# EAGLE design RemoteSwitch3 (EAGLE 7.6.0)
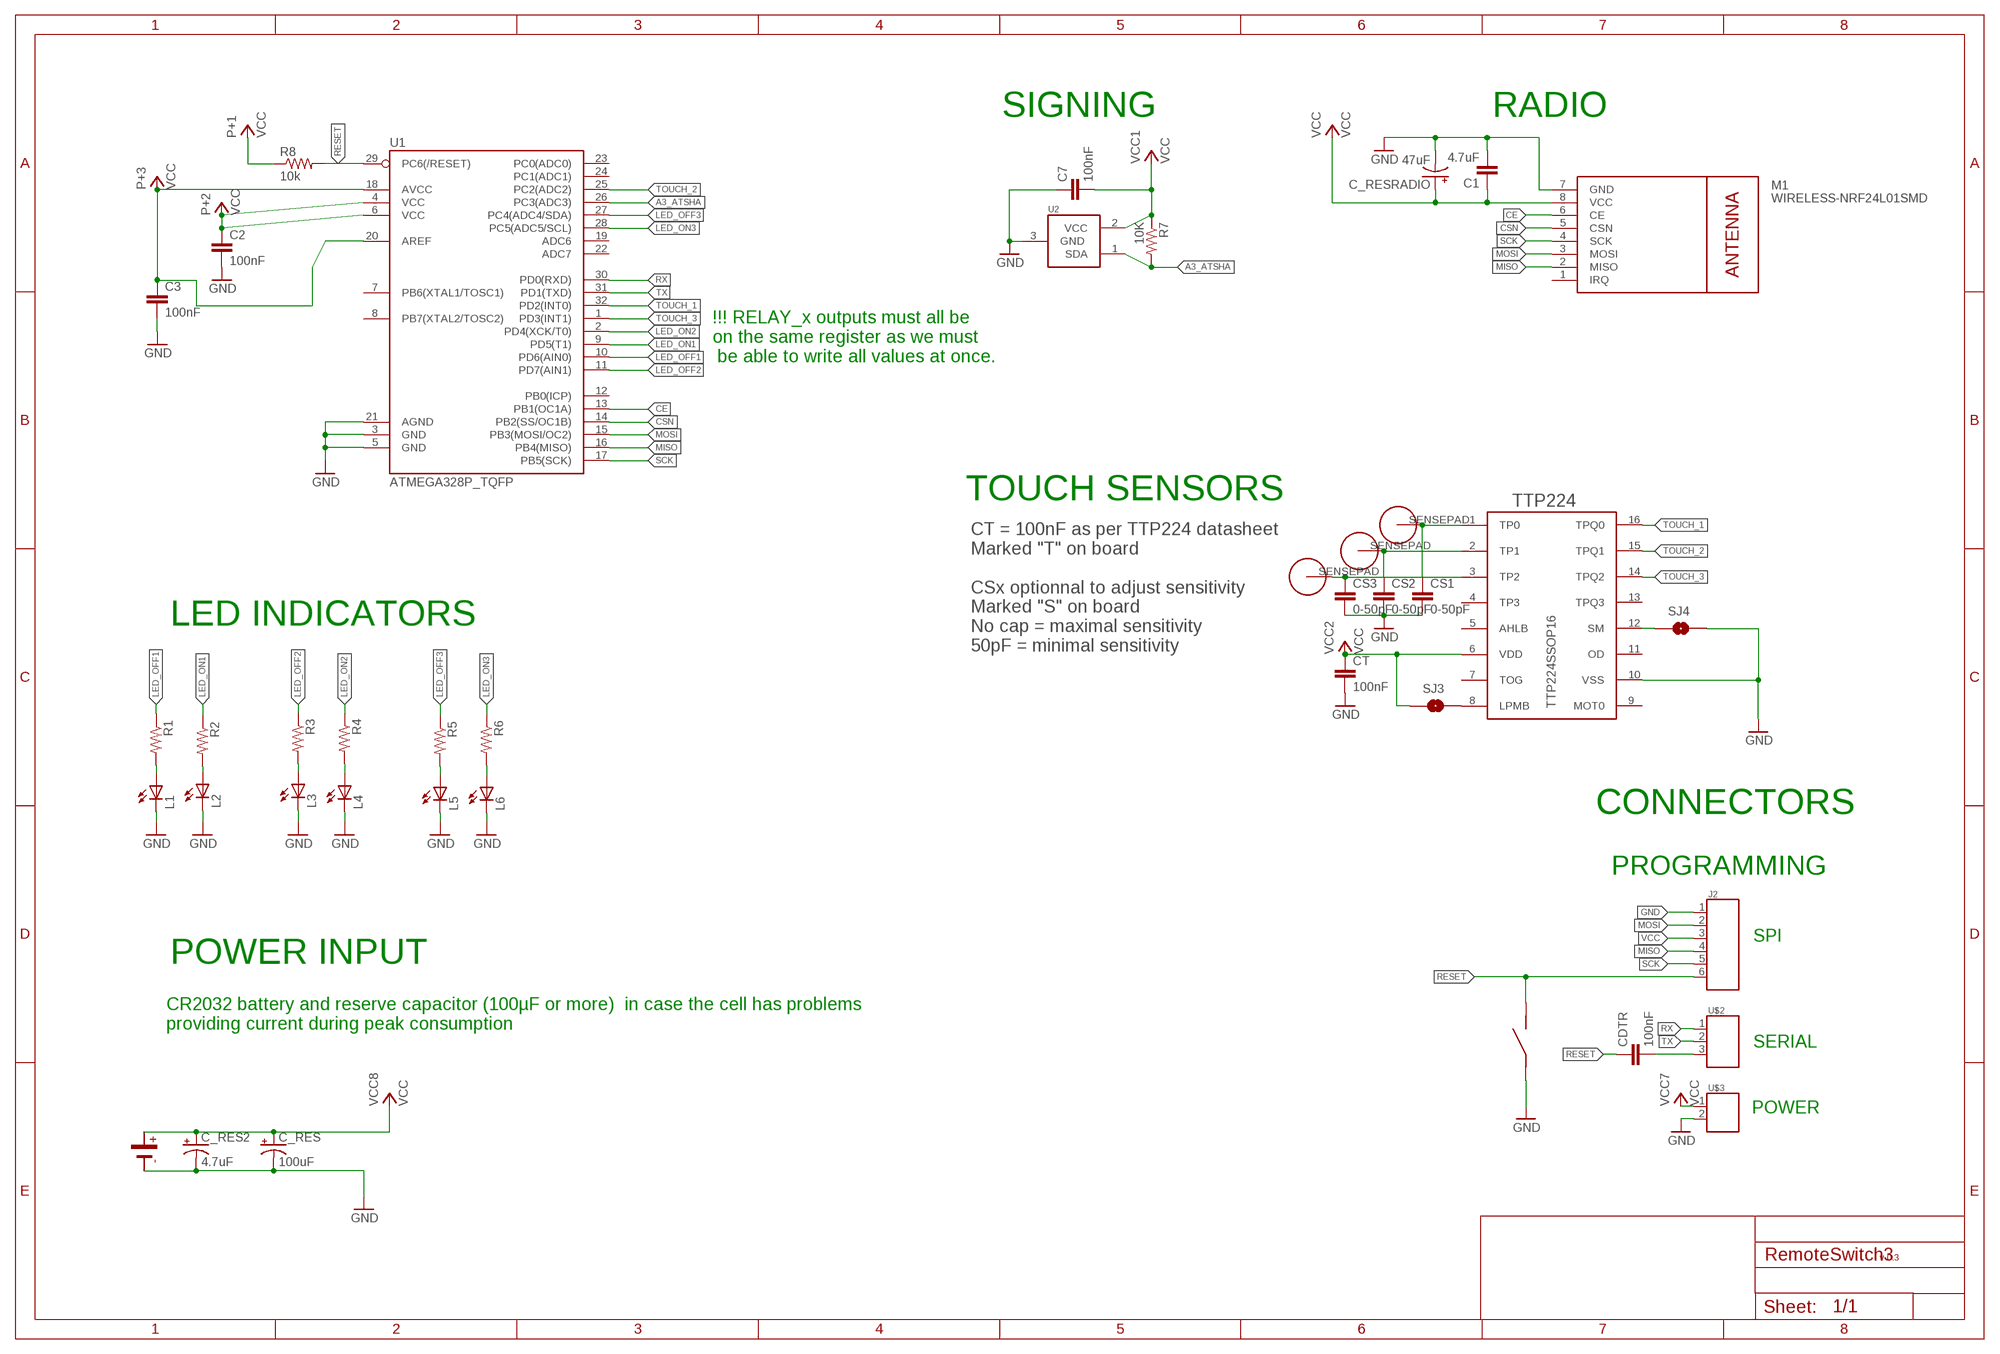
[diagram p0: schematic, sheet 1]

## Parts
C1  4.7uF  4.7UF-16V-20%,+80%-(1206)  [1206-CAP]
C2  100nF  CAP0805  [0805]
C3  100nF  CAP0805  [0805]
C7  100nF  CAP0805  [0805]
C_RES  100uF  10UF-16V-10%(TANT)  [EIA3216]
C_RES2  4.7uF  10UF-16V-10%(TANT)  [EIA3216]
C_RESRADIO  47uF  10UF-16V-10%(TANT)  [EIA3216]
CDTR  100nF  CAP0805  [0805]
CR2032  BATCR20328_SMDROUND  [BAT_CR2032_SMDROUND]
CS1  0-50pF  CAP0805  [0805]
CS2  0-50pF  CAP0805  [0805]
CS3  0-50pF  CAP0805  [0805]
CT  100nF  CAP0805  [0805]
J2  CONNECTOR_6DUP_2_3  [DUPONT_2_3]
L1  LED  [LED_0805]
L2  LED  [LED_0805]
L3  LED  [LED_0805]
L4  LED  [LED_0805]
L5  LED  [LED_0805]
L6  LED  [LED_0805]
M1  WIRELESS-NRF24L01SMD  [WIRELESS-NRF24L01-SMD]
PAD1  TOUCH_PADRECT  [TOUCH_PAD_RECT]
PAD2  TOUCH_PADRECT  [TOUCH_PAD_RECT]
PAD3  TOUCH_PADRECT  [TOUCH_PAD_RECT]
R1  RESISTOR0805-RES  [0805]
R2  RESISTOR0805-RES  [0805]
R3  RESISTOR0805-RES  [0805]
R4  RESISTOR0805-RES  [0805]
R5  RESISTOR0805-RES  [0805]
R6  RESISTOR0805-RES  [0805]
R7  10K  RESISTOR0805-RES  [0805]
R8  10k  RESISTOR0805-RES  [0805]
SJ3  JUMPER-PAD-2-NOYES_SILK  [PAD-JUMPER-2-NO_YES_SILK]
SJ4  JUMPER-PAD-2-NOYES_SILK  [PAD-JUMPER-2-NO_YES_SILK]
TTP224  TTP224SSOP16  [SSOP16]
U1  ATMEGA328P_TQFP  [TQFP32-08]
U2  IC_ATSHA204A_CRYPT  [SOT23-3]
U$1  SWITCHPROMINI_RESET  [SWITCH_SMD_PROMINI_RESET]
U$2  CONNECTOR_3DUPONT  [DUPONT_3]
U$3  CONNECTOR_2DUPONT  [DUPONT_2]

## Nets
A3_ATSHA: R7.2 U1.26(PC3(ADC3)) U2.1(SDA)
CE: M1.6(CE) U1.13(PB1(OC1A))
CSN: M1.5(CSN) U1.14(PB2(SS/OC1B))
GND: C1.2 C2.2 C3.2 C7.1 C_RES2.C(-) C_RES.C(-) C_RESRADIO.C(-) CR2032.- CS1.2 CS2.2 CS3.2 CT.2 J2.1 L1.2(C) L2.2(C) L3.2(C) L4.2(C) L5.2(C) L6.2(C) M1.7(GND) SJ4.2 TTP224.10(VSS) U1.3(GND) U1.5(GND) U1.21(AGND) U2.3(GND) U$1.IN U$3.2
LED_OFF1: R1.1 U1.10(PD6(AIN0))
LED_OFF2: R3.1 U1.11(PD7(AIN1))
LED_OFF3: R5.1 U1.27(PC4(ADC4/SDA))
LED_ON1: R2.1 U1.9(PD5(T1))
LED_ON2: R4.1 U1.2(PD4(XCK/T0))
LED_ON3: R6.1 U1.28(PC5(ADC5/SCL))
MISO: J2.4 M1.2(MISO) U1.16(PB4(MISO))
MOSI: J2.2 M1.3(MOSI) U1.15(PB3(MOSI/OC2))
N$1: L5.1(A) R5.2
N$2: CS1.1 PAD1.SENSEPAD TTP224.1(TP0)
N$3: L1.1(A) R1.2
N$4: CS2.1 PAD2.SENSEPAD TTP224.2(TP1)
N$5: CS3.1 PAD3.SENSEPAD TTP224.3(TP2)
N$6: L2.1(A) R2.2
N$8: L6.1(A) R6.2
N$9: L3.1(A) R3.2
N$10: L4.1(A) R4.2
N$11: CDTR.2 U$2.3
N$18: SJ4.1 TTP224.12(SM)
N$19: SJ3.2 TTP224.8(LPMB)
RESET: CDTR.1 J2.6 R8.2 U1.29(PC6(/RESET)) U$1.OUT
RX: U1.30(PD0(RXD)) U$2.1
SCK: J2.5 M1.4(SCK) U1.17(PB5(SCK))
TOUCH_1: TTP224.16(TPQ0) U1.32(PD2(INT0))
TOUCH_2: TTP224.15(TPQ1) U1.25(PC2(ADC2))
TOUCH_3: TTP224.14(TPQ2) U1.1(PD3(INT1))
TX: U1.31(PD1(TXD)) U$2.2
VCC: C1.1 C2.1 C3.1 C7.2 C_RES2.A(+) C_RES.A(+) C_RESRADIO.A(+) CR2032.+1(+) CR2032.+2(+) CT.1 J2.3 M1.8(VCC) R7.1 R8.1 SJ3.1 TTP224.6(VDD) U1.4(VCC) U1.6(VCC) U1.18(AVCC) U1.20(AREF) U2.2(VCC) U$3.1
Unconnected: M1.1(IRQ) TTP224.4(TP3) TTP224.5(AHLB) TTP224.7(TOG) TTP224.9(MOT0) TTP224.11(OD) TTP224.13(TPQ3) U1.7(PB6(XTAL1/TOSC1)) U1.8(PB7(XTAL2/TOSC2)) U1.12(PB0(ICP)) U1.19(ADC6) U1.22(ADC7) U1.23(PC0(ADC0)) U1.24(PC1(ADC1))

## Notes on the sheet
- SIGNING | RADIO
- !!! RELAY_x outputs must all be 
  on the same register as we must
   be able to write all values at once.
- TOUCH SENSORS
- LED INDICATORS
- CT = 100nF as per TTP224 datasheet
  Marked "T" on board
  
  CSx optionnal to adjust sensitivity
  Marked "S" on board
  No cap = maximal sensitivity
  50pF = minimal sensitivity
- CONNECTORS
- PROGRAMMING
- SPI
- POWER INPUT
- CR2032 battery and reserve capacitor (100µF or more)  in case the cell has problems
  providing current during peak consumption
- SERIAL
- POWER
- v 0.3

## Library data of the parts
C1 = SparkFun-Capacitors:4.7UF-16V-20%,+80%-(1206): CAP-10300; PROD_ID: CAP-10300
C2 C3 C7 CDTR CS1-CS3 CT = SparkFun-Passives:CAP: Capacitor
C_RES C_RES2 C_RESRADIO = SparkFun-Capacitors:10UF-16V-10%(TANT): CAP-00811; PROD_ID: CAP-00811; VALUE: 10uF
CR2032 = NCA_Sensors:BAT
J2 = TD-MySensors:CONNECTOR_6
L1-L6 = TD-MySensors:LED
M1 = nrf24l01plus:WIRELESS-NRF24L01: 2.4 GHz Wireless Module based on NRF24L01 chip
PAD1-PAD3 = NCA_Sensors:TOUCH_PAD
R1-R8 = SparkFun-Passives:RESISTOR: Resistor
SJ3 SJ4 = TD-MySensors:JUMPER-PAD-2-NO
TTP224 = NCA_Sensors:TTP224
U1 = SparkFun-DigitalIC:ATMEGA328P_TQFP; PROD_ID: IC-09069
U2 = TD-MySensors:IC_ATSHA204A_CRYPT
U$1 = NCA_Sensors:SWITCH
U$2 = TD-MySensors:CONNECTOR_3
U$3 = TD-MySensors:CONNECTOR_2: 2 Pin connector

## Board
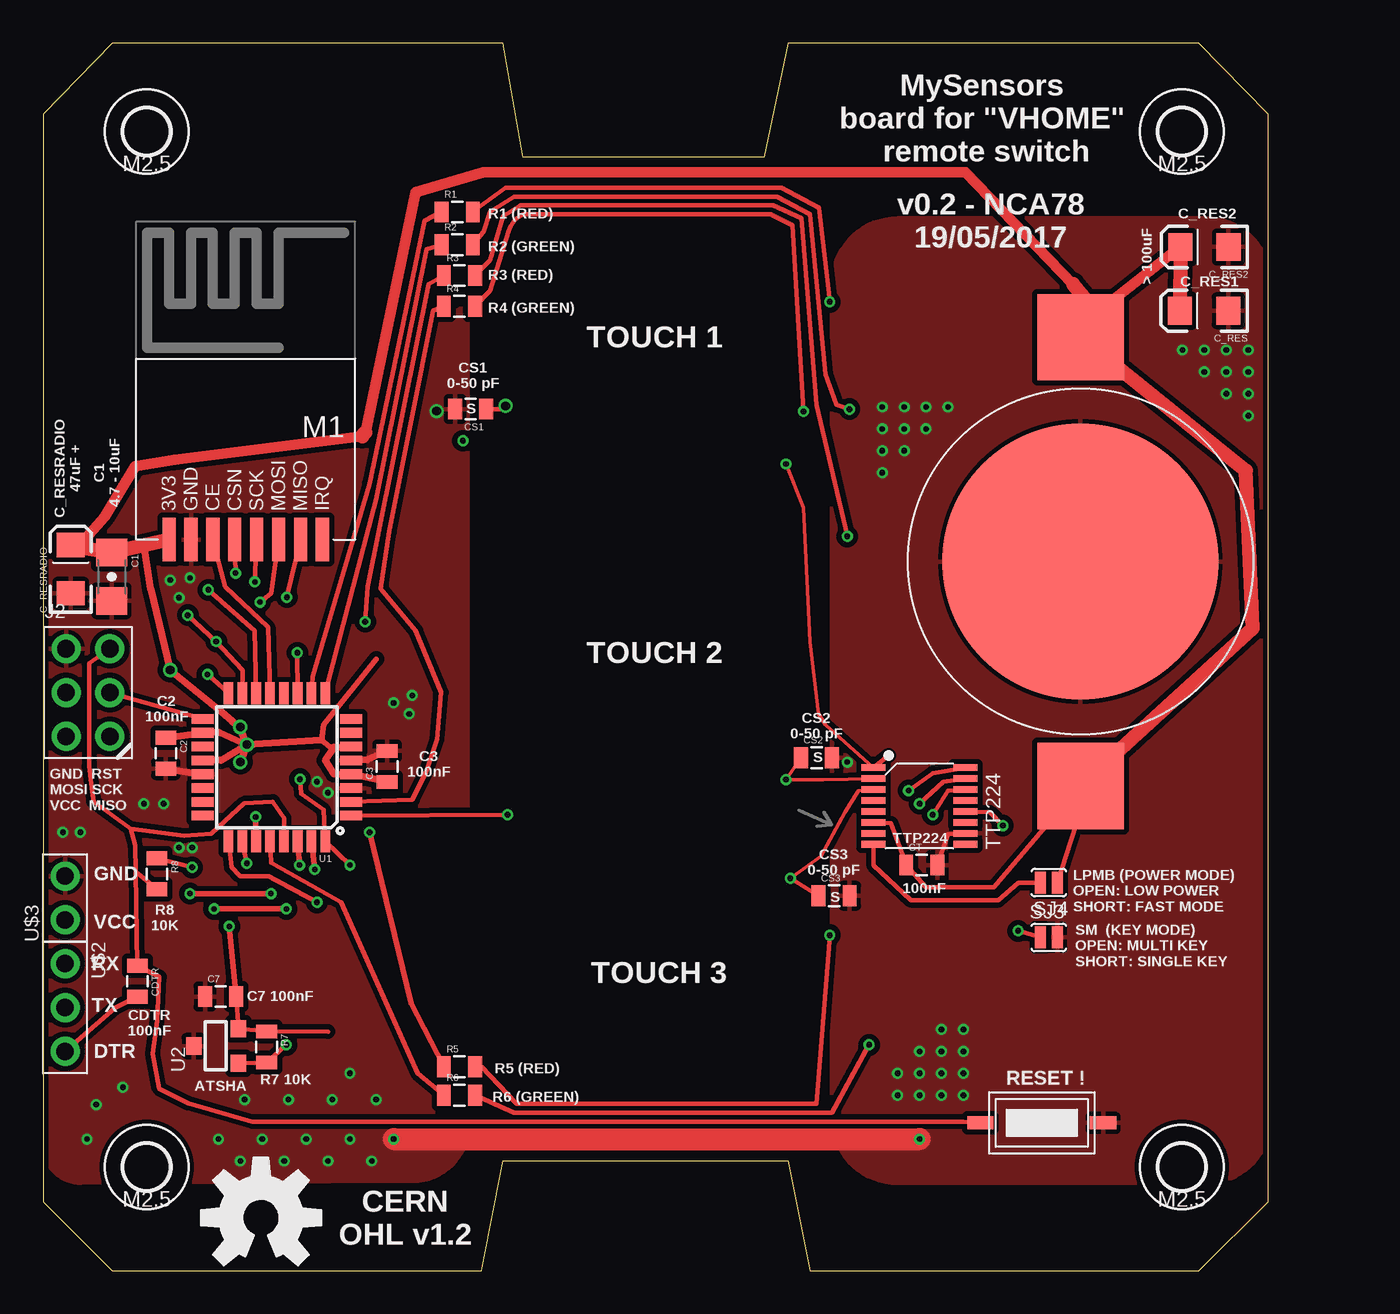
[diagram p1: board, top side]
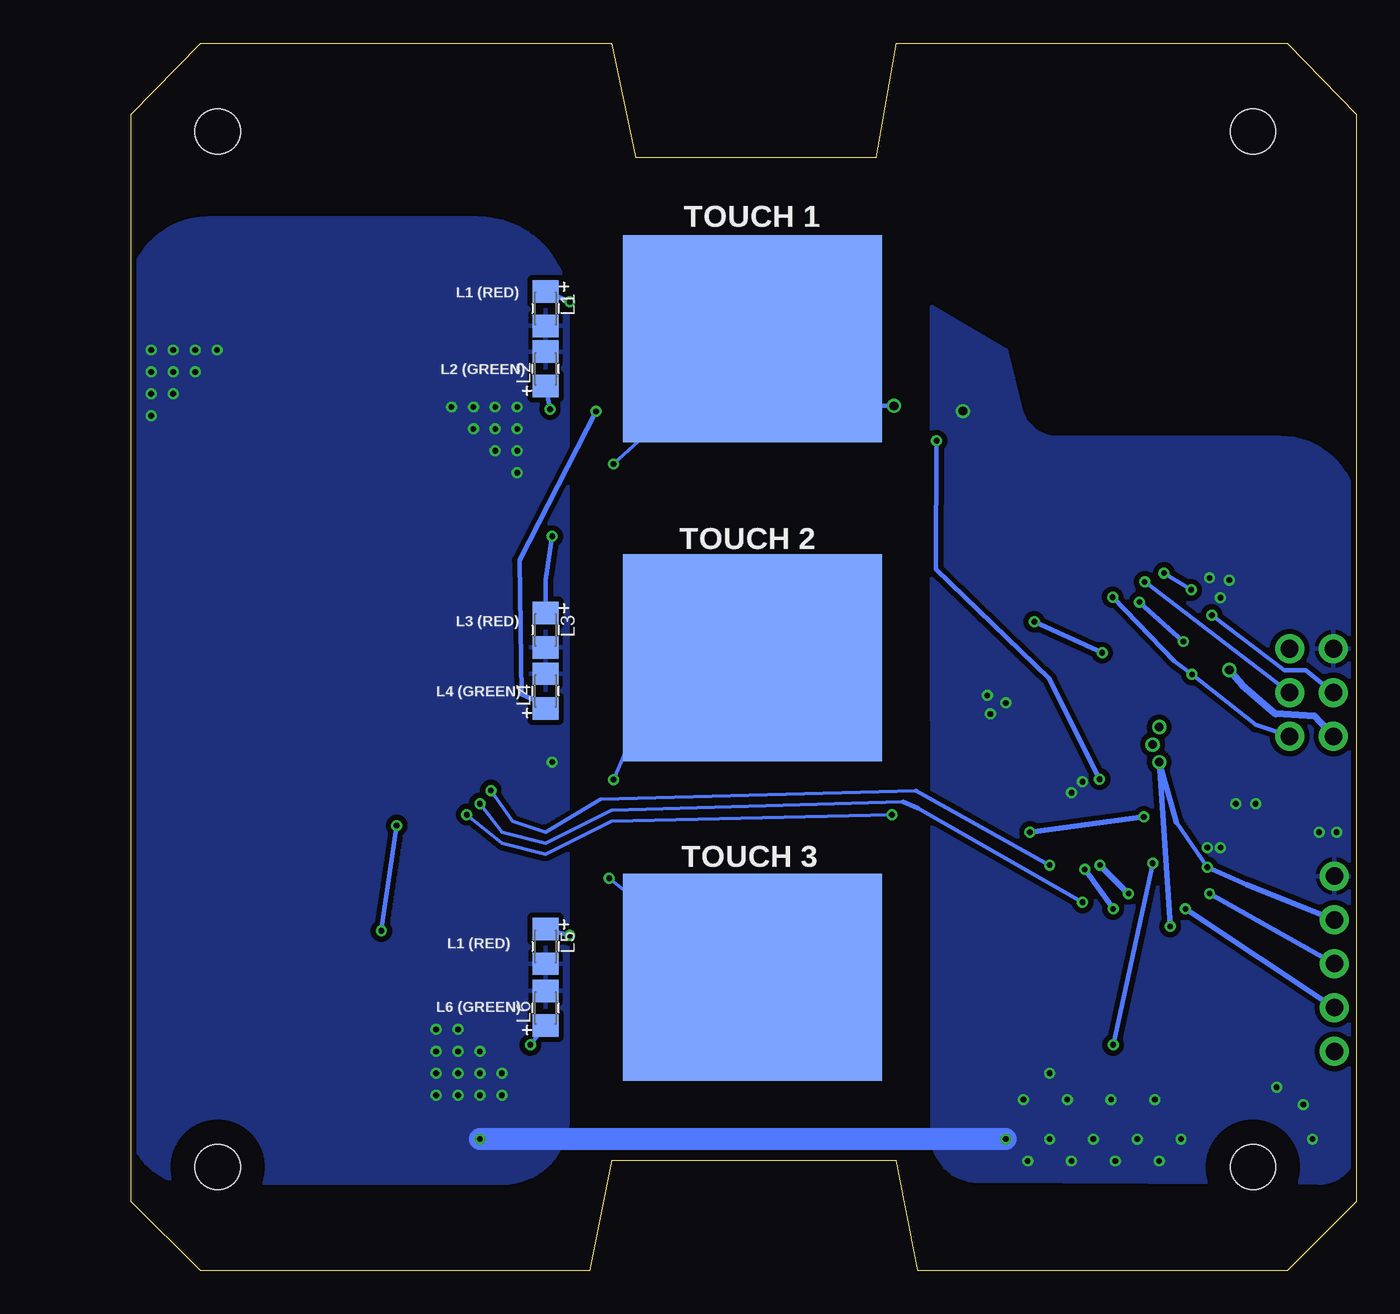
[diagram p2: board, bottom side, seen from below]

Size 71 x 71.12 mm. Coordinates in mm from the lower left corner, seen from the top.
Outline: 0,4 4,0 25.4,0 26.67,6.35 43.18,6.35 44.45,0 67,0 71,4 71,67 67,71.12 43.18,71.12 41.78,64.52 27.81,64.52 26.67,71.12 4,71.12 0,67 0,4
Copper layers (1*16): Top 0.035mm / dielectric 1.5mm / Bottom 0.035mm
Design rules "SeeedStudio_2layer_DRU_no_angle_20140221": minimum track width 6mil, minimum drill 12mil, track to track 6mil, track to pad 6mil, pad to pad 6mil, via to via 6mil, smd to smd 0mil, copper to edge 10mil, drill to drill 10mil, minimum pad ring 10mil, minimum via ring 6mil, stop-mask expansion 2mil, vias tented up to drill 100mil, thermal gap 10mil

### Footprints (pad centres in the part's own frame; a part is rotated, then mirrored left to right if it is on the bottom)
1206-CAP = smd 1.6 x 1.8: 1 -1.4,0; 2 1.4,0
0805 = smd 0.8 x 1.2: 1 -0.9,0; 2 0.9,0
EIA3216 = smd 1.4 x 1.6: A 1.4,0; C -1.4,0
BAT_CR2032_SMDROUND = smd 5 x 5: +1 13,0; +2 -13,0 | smd 16 x 16: - 0,0
DUPONT_2_3 = drill 1.016 pad 1.676: 1 -1.27,2.54; 2 -1.27,0; 3 -1.27,-2.54; 4 1.27,-2.54; 5 1.27,0; 6 1.27,2.54
LED_0805 = smd 1.3 x 1.5: 1 -1,0; 2 1,0
WIRELESS-NRF24L01-SMD = smd 2.54 x 0.762: 1 1.27,0; 2 1.27,1.27; 3 1.27,2.54; 4 1.27,3.81; 5 1.27,5.08; 6 1.27,6.35; 7 1.27,7.62; 8 1.27,8.89
TOUCH_PAD_RECT = smd 15 x 12: SENSEPAD 0,0
PAD-JUMPER-2-NO_YES_SILK = smd 0.635 x 1.27: 1 -0.501,0; 2 0.501,0
SSOP16 = smd 0.381 x 1.397: 1 0.318,-0.762; 2 0.953,-0.762; 3 1.587,-0.762; 4 2.223,-0.762; 5 2.857,-0.762; 6 3.493,-0.762; 7 4.128,-0.762; 8 4.763,-0.762; 9 4.763,4.572; 10 4.128,4.572; 11 3.493,4.572; 12 2.857,4.572; 13 2.223,4.572; 14 1.587,4.572; 15 0.953,4.572; 16 0.318,4.572
TQFP32-08 = smd 1.27 x 0.559: 1 -4.293,2.8; 2 -4.293,2; 3 -4.293,1.2; 4 -4.293,0.4; 5 -4.293,-0.4; 6 -4.293,-1.2; 7 -4.293,-2; 8 -4.293,-2.8; 17 4.293,-2.8; 18 4.293,-2; 19 4.293,-1.2; 20 4.293,-0.4; 21 4.293,0.4; 22 4.293,1.2; 23 4.293,2; 24 4.293,2.8 | smd 0.559 x 1.27: 9 -2.8,-4.293; 10 -2,-4.293; 11 -1.2,-4.293; 12 -0.4,-4.293; 13 0.4,-4.293; 14 1.2,-4.293; 15 2,-4.293; 16 2.8,-4.293; 25 2.8,4.293; 26 2,4.293; 27 1.2,4.293; 28 0.4,4.293; 29 -0.4,4.293; 30 -1.2,4.293; 31 -2,4.293; 32 -2.8,4.293
SOT23-3 = smd 1 x 0.9: 1 -1,-1.3; 2 1,-1.3; 3 0,1.3
SWITCH_SMD_PROMINI_RESET = smd 1.524 x 0.762: IN -0.508,1.778; OUT 6.604,1.778
DUPONT_3 = drill 1.016 pad 1.676: 1 -2.54,0; 2 0,0; 3 2.54,0
DUPONT_2 = drill 1.016 pad 1.676: 1 -1.27,0; 2 1.27,0
HOLE_M2.5PAN_TIGHT = hole 2.6: 0,0

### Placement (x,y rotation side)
C1  3.97,40.2 270 top
C2  7.11,29.97 270 top
C3  19.94,29.21 90 top
C7  10.29,15.88 0 top
C_RES  67.29,55.62 180 top
C_RES2  67.31,59.31 180 top
C_RESRADIO  1.6,40.64 90 top
CDTR  5.46,16.76 270 top
CR2032  60.13,41.08 90 top
CS1  24.77,49.92 180 top
CS2  44.83,29.72 0 top
CS3  45.85,21.72 0 top
CT  50.93,23.5 0 top
J2  2.6,33.49 0 top
L1  47,55.74 270 bottom
L2  47,52.25 90 bottom
L3  47,37.11 270 bottom
L4  47,33.58 90 bottom
L5  47,18.78 270 bottom
L6  47,15.21 90 bottom
M1  16.19,41.09 90 top
PAD1  35,54 0 bottom
PAD2  35,35.5 0 bottom
PAD3  35,17 0 bottom
R1  24,61.34 0 top
R2  24,59.44 0 top
R3  24.13,57.66 0 top
R4  24.13,55.88 0 top
R5  24.13,11.81 0 top
R6  24.13,10.16 0 top
R7  12.95,12.95 270 top
R8  6.6,22.99 270 top
SJ3  58.29,22.48 180 top
SJ4  58.29,19.3 0 top
TTP224  48.9,29.46 270 top
U1  13.55,29.16 180 top
U2  10.03,13.01 90 top
U$1  60.94,10.34 180 top
U$2  1.27,15.24 270 top
U$3  1.27,21.59 90 top
U$4  [OSHW-LOGO-L]  12.63,3.07 0 top
U$5  [HOLE_M2.5PAN_TIGHT]  6,66 0 top
U$6  [HOLE_M2.5PAN_TIGHT]  6,6 0 top
U$7  [HOLE_M2.5PAN_TIGHT]  66,6 0 top
U$8  [HOLE_M2.5PAN_TIGHT]  66,66 0 top

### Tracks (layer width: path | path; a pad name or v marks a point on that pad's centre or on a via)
A3_ATSHA  (via drill 0.33)
  Top 0.254: U2.1 R7.2 v14.1,13.08 | v11.8,23.6 U1.26
  Bottom 0.254: v11.8,23.6 v14.1,13.08
CE
  Top 0.254: M1.6 10.54,39.62 13.03,37.26 U1.13
CSN  (via drill 0.33)
  Top 0.254: U1.14 12.27,37.08 v9.58,39.45 | v11.15,40.41 M1.5
  Bottom 0.254: v9.58,39.45 v11.15,40.41
GND  (via drill 0.33, 0.51)
  Top 0.254: CT.2 52.45,25.27 TTP224.10
  Top 0.406: C2.2 U1.21 | C3.2 18.8,29.59 U1.5
  Top 1.27: v20.32,7.62 v50.8,7.62
  Bottom 1.27: v20.32,7.62 v50.8,7.62
  other vias: 52.07,11.43 49.53,11.43 49.53,10.16 50.8,11.43 50.8,12.7 53.34,12.7 52.07,12.7 2.54,7.62 3.08,9.62 17.78,7.62 15.24,7.62 12.7,7.62 10.16,7.62 4.62,10.62 1.14,25.4 2.16,25.4 7.37,40.01 7.87,38.99 8.51,40.13 15.88,28.32 16.51,27.69 21.39,33.32 20.32,32.89 21.21,32.26 5.84,27.05 6.99,27.05 50.8,10.16 52.07,10.16 53.34,11.43 53.34,10.16 52.07,13.97 53.34,13.97 46.61,29.46 14.22,9.91 16.76,9.91 11.68,9.91 19.3,9.91 48.64,50.04 49.91,50.04 51.18,50.04 52.45,50.04 51.18,48.77 49.91,48.77 48.64,48.77 48.64,47.5 49.91,47.5 48.64,46.23 8.64,24.51 7.87,24.51 66.04,53.34 67.31,53.34 68.58,53.34 69.85,53.34 69.85,52.07 68.58,52.07 67.31,52.07 68.58,50.8 69.85,50.8 69.85,49.53 11.43,6.35 13.97,6.35 16.51,6.35 19.05,6.35 17.78,11.43 22.8,49.8
  pour Top (isolate 0.305): 67.44,60.96 49.54,60.96 arc90 45.72,57.14 45.72,8.88 arc90 49.52,5.08 67.46,5.08 arc90 71.12,8.74 71.12,57.28 arc90
  pour Top (isolate 0.305): 24.61,56.01 21.79,54.26 arc44 19.9,51.66 19.46,49.91 arc-76 17.35,48.26 3.76,48.26 arc90 0,44.5 0,7.29 arc90 2.21,5.09 21.46,5.19 arc90 24.61,8.36
  pour Bottom (isolate 0.305): 24.61,55.85 20.32,53.34 19.46,49.91 arc-76 17.35,48.26 4.43,48.26 arc90 0,43.83 0,7.29 arc90 2.21,5.09 21.9,5.19 arc90 24.56,7.87
  pour Bottom (isolate 0.305): 66.56,60.96 50.92,60.96 arc90 45.72,55.76 45.72,8.88 arc90 49.52,5.08 67.46,5.08 arc90 71.12,8.74 71.12,56.4 arc90
LED_OFF1
  Top 0.254: U1.10 15.62,34.42 18.92,45.59 22.1,60.83 R1.1
LED_OFF2  (via drill 0.33)
  Top 0.254: v14.73,35.8 U1.11 | R3.1 22.35,57.15 18.8,39.62 v18.67,37.59
  Bottom 0.254: v18.67,37.59 v14.73,35.8
LED_OFF3  (via drill 0.33)
  Top 0.305: R5.1 21.34,15.49 v18.92,25.4 | v12.32,26.29 U1.27
  Bottom 0.305: v18.92,25.4 v12.32,26.29
LED_ON1
  Top 0.254: R2.1 22.23,59.18 19.3,44.7 U1.9
LED_ON2
  Top 0.254: U1.2 21.4,27.28 22.19,28.88 22.82,30.78 23.08,33.5 21.59,37.08 19.56,39.5 20.07,42.8 22.61,55.63 R4.1
LED_ON3
  Top 0.254: U1.28 13.21,23.62 17.27,21.34 21.71,11.43 R6.1
MISO  (via drill 0.33)
  Top 0.254: M1.2 v14.12,39.01 | v9.53,34.54 U1.16
  Bottom 0.254: v14.12,39.01 10.54,35.31 v9.53,34.54 5.84,31.62 J2.4
MOSI  (via drill 0.33)
  Top 0.254: M1.3 13.21,39.24 v12.57,38.73 | v8.38,37.97 v10.03,36.45 11.56,34.8 U1.15
  Bottom 0.254: J2.2 2.92,34.8 4.19,34.8 v8.38,37.97 | v10.03,36.45 v12.57,38.73
N$1  (via drill 0.33)
  Top 0.254: R5.2 25.4,11.81 27.43,9.65 44.83,9.65 v45.59,19.43
  Bottom 0.254: v45.59,19.43 L5.1
N$2  (via drill 0.33, 0.51)
  Top 0.203: TTP224.1 45.34,31.62 44.94,32.27 44.45,36.45 44.07,44.2 v43.05,46.74
  Top 0.254: 49.02,29.84 TTP224.1 | CS1.1 26.62,49.92 v26.8,50.1
  Bottom 0.203: v43.05,46.74 PAD1.SENSEPAD
  Bottom 0.254: v26.8,50.1 31.1,50.1 PAD1.SENSEPAD
N$3  (via drill 0.33)
  Top 0.254: R1.2 26.8,62.74 42.8,62.74 44.96,61.59 v45.59,56.13
  Bottom 0.254: v45.59,56.13 L1.1
N$4  (via drill 0.33)
  Top 0.203: CS2.1 v43.05,28.45 45.21,28.45 TTP224.2
  Bottom 0.203: v43.05,28.45 42.1,30.67 41.78,30.99
  Bottom 0.254: PAD2.SENSEPAD 42.1,30.67
N$5  (via drill 0.33)
  Top 0.203: CS3.1 v43.31,22.73 45.09,24 46.48,26.54 47.24,27.81 TTP224.3
  Bottom 0.203: v43.31,22.73 41.91,21.59
  Bottom 0.254: PAD3.SENSEPAD 41.91,21.59
N$6  (via drill 0.33)
  Top 0.254: R2.2 25.53,60.2 25.91,61.34 27.3,62.23 42.55,62.23 44.45,61.21 45.34,51.94 45.97,50.16 v46.74,49.91
  Bottom 0.254: v46.74,49.91 L2.1
N$8  (via drill 0.33)
  Top 0.254: R6.2 27.3,9.14 45.72,9.14 v47.88,13.08
  Bottom 0.254: v47.88,13.08 L6.1
N$9  (via drill 0.33)
  Top 0.254: R3.2 25.91,58.55 26.67,61.09 27.69,61.72 42.29,61.72 43.94,60.96 44.83,50.16 v46.61,42.55
  Bottom 0.254: L3.1 46.99,40.01 v46.61,42.55
N$10  (via drill 0.33)
  Top 0.254: R4.2 25.91,56.77 26.99,60.23 arc-42 27.72,61.16 27.81,61.21 42.16,61.21 43.43,60.58 v44.07,49.78
  Bottom 0.254: v44.07,49.78 48.51,41.15 48.39,33.4 46.74,32.64 L4.1
N$11
  Top 0.254: U$2.3 4.19,15.24 CDTR.2
N$18  (via drill 0.33)
  Top 0.254: TTP224.12 54.86,26.54 v55.63,25.78 | v56.52,19.68 SJ4.1
  Bottom 0.254: v55.63,25.78 v56.52,19.68
N$19
  Top 0.254: TTP224.8 48.13,23.5 50.29,21.46 55.37,21.46 56.52,22.48 SJ3.2
RESET
  Top 0.254: U1.29 13.97,26.21 13.31,27.18 11.66,27.08 9.73,25.32 8.17,25.19 5.09,25.6 | J2.6 2.67,35.18 2.67,29.21 2.82,27.98 2.92,27.18 5.09,25.6 | 5.09,25.6 5.33,24.64 5.36,23.11 | 5.36,23.11 CDTR.1 6.73,17.02 6.6,14.48 6.35,12.57 6.73,10.54 8.4,9.7 12.13,8.64 53.34,8.64 U$1.OUT | R8.2 5.36,23.11
RX  (via drill 0.33)
  Top 0.305: v8.51,21.84 v13.21,21.84 | v14.86,23.5 U1.30
  Bottom 0.305: U$2.1 v8.51,21.84 | v13.21,21.84 v14.86,23.5
SCK  (via drill 0.33)
  Top 0.254: M1.4 v12.27,39.9 | J2.5 U1.17
  Bottom 0.254: v12.27,39.9 J2.5
TOUCH_1  (via drill 0.33)
  Top 0.254: v14.88,28.47 14.96,27.64 16.26,26.7 U1.32 v17.78,23.5 | TTP224.16 51.56,28.83 v50.16,27.81
  Bottom 0.203: v50.16,27.81 48.9,26.04 46.99,25.4 43.81,27.3 25.53,27.81
  Bottom 0.254: v24.33,48.08 24.38,40.64 17.78,34.29 v14.88,28.47 | 25.53,27.81 v17.78,23.5
TOUCH_2  (via drill 0.33)
  Top 0.254: v15.88,21.34 13.08,22.86 11.43,22.86 10.92,23.37 U1.25 | TTP224.15 52.2,28.32 v50.8,27.05
  Bottom 0.203: v50.8,27.05 49.53,25.4 46.99,24.77 43.18,26.67 26.29,27.18
  Bottom 0.254: v15.88,21.34 25.4,26.8 26.29,27.18
TOUCH_3  (via drill 0.33)
  Top 0.254: TTP224.14 52.45,27.81 v51.56,26.42 | v26.92,26.42 U1.1
  Bottom 0.203: v51.56,26.42 49.53,24.77 46.99,24.13 43.18,26.04 v26.92,26.42
TX  (via drill 0.33)
  Top 0.305: U1.31 v15.75,23.24 | v14.1,20.95 v9.91,20.95
  Bottom 0.305: v15.75,23.24 v14.1,20.95 | v9.91,20.95 U$2.2
VCC  (via drill 0.33, 0.51)
  Top 0.254: C7.2 U2.2 R7.1 16.51,13.84 | R8.1 v8.64,23.37 | CR2032.+2 55.12,22.23 51.18,22.23 CT.1 49.15,25.91 TTP224.6 | SJ3.1 60.96,29.21 61.14,29.01
  Top 0.305: C7.2 v10.79,19.94 | 19.3,35.43 16.26,31.62 16.13,30.73 16.79,30.21
  Top 0.406: C2.1 U1.18 10.21,31.19 v11.81,30.48 | C3.1 U1.4 16.84,28.78 16.36,29.57 16.79,30.21 16.87,30.33 U1.6 | U1.20 10.31,29.57 v11.81,30.48 | C1.1 5.84,42.16 6.22,39.5 v7.37,34.8 10.16,32.51 10.94,31.87 v11.43,31.5 v11.81,30.48 | v11.81,30.48 v11.43,29.46 | 16.13,30.73 v11.81,30.48
  Top 0.61: 18.49,48.34 7.62,46.99 5.33,46.61 3.56,43.69 2.04,41.95 | 18.68,48.57 21.59,62.48 25.53,63.63 53.47,63.63 59.69,57.15 | C_RES2.A 61.09,55.5
  Top 0.813: C_RESRADIO.A 2.04,41.95 C1.1 M1.8 | 18.49,48.34 18.68,48.57 | 59.69,57.15 61.09,55.5 CR2032.+1 69.72,46.35 70.1,37.21 61.14,29.01 CR2032.+2 | C_RES2.A C_RES.A
  Bottom 0.254: 10.43,25.97 v8.64,23.37 6.35,22.35
  Bottom 0.305: v10.79,19.94 v11.43,29.46 10.43,25.97 | U$3.1 6.35,22.35
  Bottom 0.406: J2.3 2.41,32.13 4.7,32.26 6.6,33.91 v7.37,34.8

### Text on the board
tPlace: MySensors / board for "VHOME" / remote switch | R1 (RED) | C_RES2 | v0.2 - NCA78 / 19/05/2017 | R2 (GREEN) | R3 (RED) | > 100uF | C_RES1 | R4 (GREEN) | TOUCH 1 | CS1 / 0-50 pF | S | C_RESRADIO / 47uF + | C1 / 4.7 - 10uF | TOUCH 2 | C2 / 100nF | CS2 / 0-50 pF | S | C3 / 100nF | GND RST / MOSI SCK / VCC MISO | TTP224 | CS3 / 0-50 pF | GND | LPMB (POWER MODE) / OPEN: LOW POWER / SHORT: FAST MODE | S | 100nF | VCC | R8 / 10K | SM (KEY MODE) / OPEN: MULTI KEY / SHORT: SINGLE KEY | RX | TOUCH 3 | C7 100nF | TX | CDTR / 100nF | DTR | R7 10K | R5 (RED) | RESET ! | ATSHA | R6 (GREEN) | CERN / OHL v1.2
bPlace: TOUCH 1 | L1 (RED) | L2 (GREEN) | TOUCH 2 | L3 (RED) | L4 (GREEN) | TOUCH 3 | L1 (RED) | L6 (GREEN)
tDocu: Minimize crossing with TOUCH 3 electrode: / 8 mil traces + perpendicular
